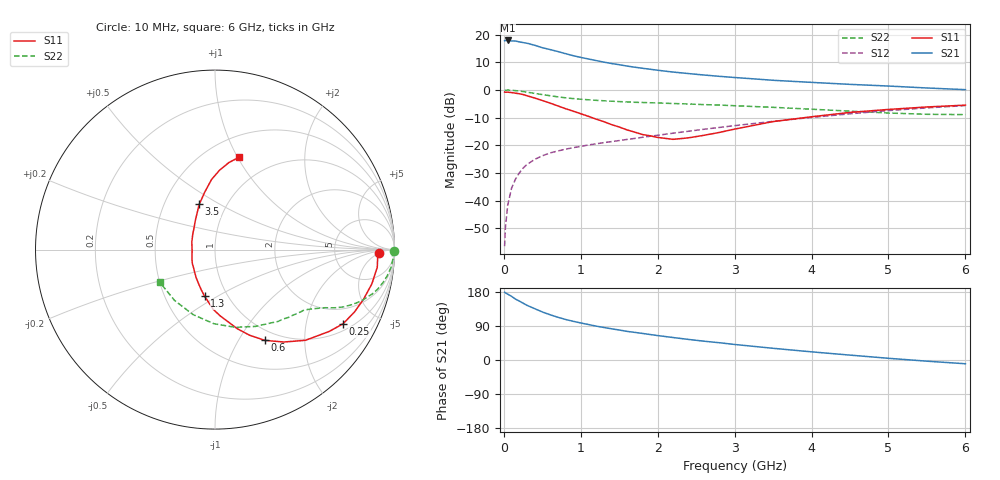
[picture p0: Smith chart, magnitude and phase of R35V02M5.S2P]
! SIEMENS Small Signal Semiconductors
! BFR181
! Si NPN RF Bipolar Junction Transistor in SOT23
! VCE = 5 V  IC = 2.5 mA
! Common Emitter S-Parameters:  May  1996
# GHz  S  MA  R  50
!  f  S11  S21  S12  S22
! GHz  MAG  ANG  MAG  ANG  MAG  ANG  MAG  ANG
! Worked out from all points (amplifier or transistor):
!   36 points, 10 MHz to 6 GHz, reference 50 ohm
!   highest |S21| = 17.9 dB at 50 MHz (marker M1)
!   |S21| within 3 dB of that: start of sweep to 558 MHz
!   unconditionally stable (mu >= 1): 1.497 GHz to 3.295 GHz
!   at 250 MHz: K = 0.26, MSG = 22.7 dB, |S12| = -28.3 dB
!   at 1.4 GHz: K = 0.98, MSG = 14.1 dB, |S12| = -18.7 dB
!   at 6 GHz: K = 0.86, MSG = 2.9 dB, |S12| = -5.7 dB
!   S11 on the Smith chart (normalised r, x): 10 MHz: 21, -5; 250 MHz: 1.26, -3.27; 600 MHz: 0.86, -1.30; 1.3 GHz: 0.78, -0.44; 3.5 GHz: 0.74, +0.40; 6 GHz: 0.71, +1.01
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0.01  0.9144 -1.2  7.736 178.8  0.0015 91.2  0.9964 -0.6
0.02  0.9074 -2.4  7.786 177.2  0.0032 85.4  0.986 -1.2
0.05  0.9094 -6.2  7.816 173.8  0.0082 87.8  0.9928 -3.0
0.1  0.8947 -12.3  7.65 168.0  0.0167 81.8  0.9858 -5.8
0.15  0.8728 -18.4  7.64 160.9  0.0242 78.6  0.9699 -8.8
0.25  0.8245 -30.1  7.154 150.0  0.0384 73.0  0.9334 -13.6
0.3  0.783 -35.6  6.97 144.3  0.0448 70.4  0.911 -15.7
0.4  0.7135 -45.1  6.405 135.6  0.0553 66.0  0.8649 -19.3
0.5  0.6422 -53.3  5.782 126.8  0.0644 62.6  0.8222 -21.9
0.6  0.5772 -61.2  5.36 119.5  0.0725 60.1  0.7846 -24.0
0.7  0.5146 -68.0  4.939 112.9  0.0785 58.5  0.7493 -25.6
0.8  0.4585 -74.2  4.522 107.1  0.0847 57.2  0.7199 -26.8
0.9  0.4128 -79.2  4.153 102.2  0.0902 56.8  0.6966 -27.7
1.1  0.3326 -91.8  3.617 93.6  0.101 56.1  0.6621 -29.6
1.3  0.2666 -102.5  3.175 85.9  0.1114 56.2  0.6354 -31.2
1.6  0.1894 -123.5  2.695 75.6  0.1273 57.1  0.6066 -33.7
2.2  0.1277 -177.8  2.099 59.3  0.165 58.0  0.5669 -40.2
2.8  0.1701 133.0  1.758 45.6  0.2094 56.9  0.5323 -48.8
3.5  0.2674 109.2  1.491 30.9  0.27 53.5  0.4838 -62.2
4.5  0.3914 92.8  1.258 12.9  0.3698 44.8  0.4127 -91.0
5.5  0.4913 80.9  1.082 -3.1  0.4729 32.5  0.362 -128.6
6  0.5301 75.6  1.009 -9.9  0.5203 25.4  0.3573 -149.3
